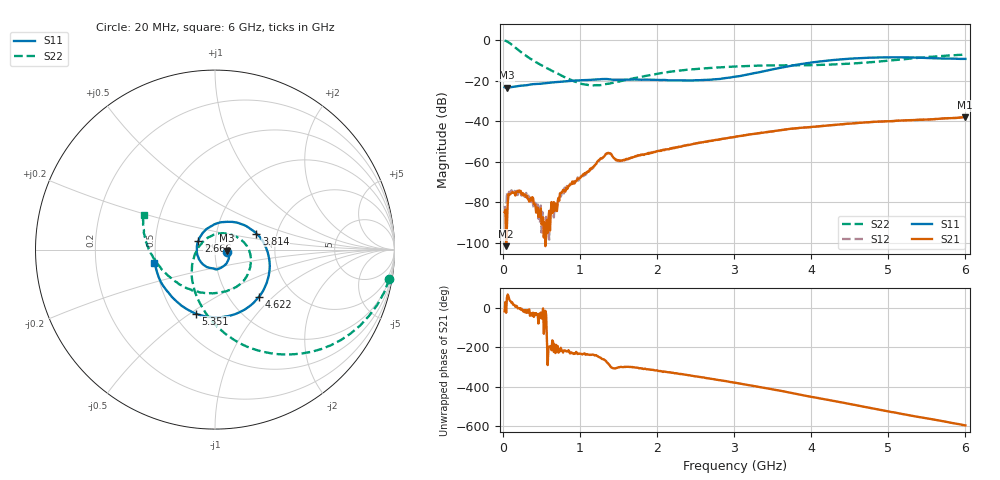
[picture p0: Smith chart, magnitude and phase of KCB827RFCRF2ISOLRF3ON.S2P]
!Agilent Technologies,E5071B,JP1KK00126,A.08.11
!Date: Tue May 06 07:30:17 2014
!Data & Calibration Information:
!Freq	S11:SOLT2(ON)	S21:SOLT2(ON)	S12:SOLT2(ON)	S22:SOLT2(ON)
# Hz S dB R 50
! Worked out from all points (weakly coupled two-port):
!   600 points, 20 MHz to 6 GHz, reference 50 ohm
!   highest |S21| = -38.03 dB at 5.99 GHz (marker M1); lowest = -101.7 dB at 39.97 MHz (marker M2)
!   lowest |S11| = -23.4 dB at 49.95 MHz (marker M3), VSWR 1.14, Z = 57.2 - j0.65 ohm
!   |S11| at or under -10 dB: start of sweep to 4.226 GHz
!   |S22| runs from -22.4 to -0.1 dB; largest |S21 - S12| = 0.00015
!   S11 on the Smith chart (normalised r, x): 20 MHz: 1.14, -0.03; 2.666 GHz: 0.83, +0.08; 3.814 GHz: 1.57, +0.30; 4.622 GHz: 1.36, -0.82; 5.351 GHz: 0.64, -0.53; 6 GHz: 0.49, -0.08
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2e7  -23.19 -12.6  -84.87 -16.6  -81.80 -11.6  -0.13 -9.6
3.996661e7  -23.39 -6.2  -101.69 -23.7  -84.00 51.6  -0.40 -18.9
4.994992e7  -23.41 -4.8  -92.13 53.6  -75.04 42.4  -0.60 -23.3
1.397997e8  -22.99 -3.9  -75.19 17.8  -75.25 14.5  -3.04 -56.0
2.196661e8  -22.52 -6.2  -75.12 -0.2  -75.00 -6.6  -5.49 -76.0
3.294825e8  -22.09 -12.6  -78.56 -10.7  -76.75 -23.2  -8.52 -95.7
4.193322e8  -21.64 -16.4  -81.25 -35.8  -80.25 -48.4  -10.68 -109.1
6.788982e8  -20.73 -33.3  -80.66 131.1  -84.40 156.2  -15.97 -143.8
7.687479e8  -20.45 -40.1  -74.77 143.0  -76.60 141.8  -17.70 -156.1
1.018331e9  -19.75 -58.6  -67.05 126.8  -67.08 124.9  -21.57 159.6
1.357763e9  -19.19 -88.4  -55.68 81.0  -55.87 80.4  -21.54 92.8
1.517496e9  -19.51 -100.5  -59.64 60.7  -59.53 59.4  -20.33 69.7
2.016661e9  -19.65 -142.5  -54.58 41.2  -54.86 42.1  -16.47 23.7
2.665576e9  -19.57 151.9  -49.84 2.8  -49.78 3.0  -13.73 -13.3
3.014992e9  -18.03 109.4  -47.72 -19.7  -47.79 -20.0  -12.98 -32.1
3.813656e9  -12.12 21.1  -43.44 -76.9  -43.45 -77.1  -12.40 -76.2
4.013322e9  -10.99 3.1  -42.79 -92.0  -42.81 -92.0  -12.31 -89.7
4.622304e9  -8.89 -47.3  -40.77 -136.8  -40.79 -136.9  -11.30 -132.8
5.011653e9  -8.46 -77.9  -39.98 -166.5  -40.02 -166.6  -10.05 -158.9
5.351085e9  -8.58 -106.6  -39.41 169.4  -39.36 169.2  -8.88 -177.8
5.990017e9  -9.25 -166.8  -38.03 124.0  -38.04 124.0  -7.12 154.8
6e9  -9.24 -167.8  -38.04 123.5  -38.04 123.2  -7.11 154.5
